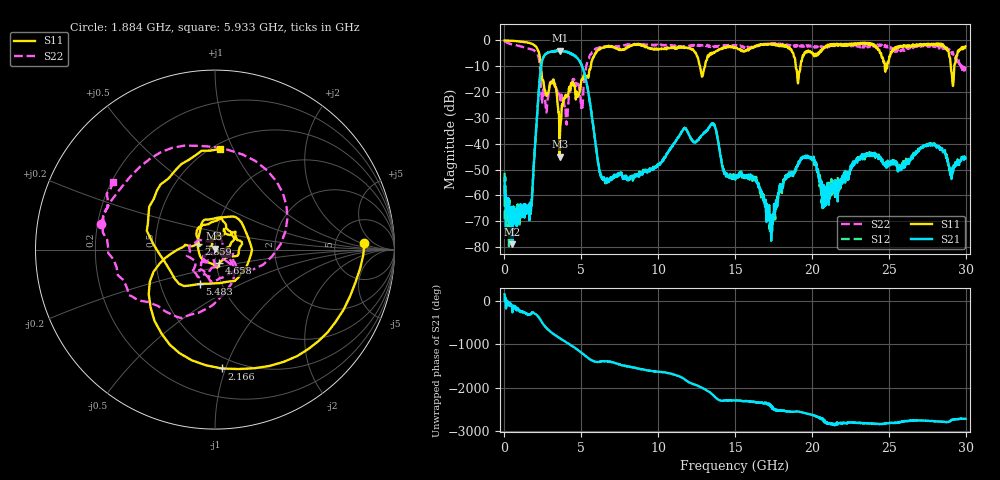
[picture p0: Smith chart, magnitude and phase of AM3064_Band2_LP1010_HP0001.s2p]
# Hz S DB R 50.0
!freq dBS11 angS11 dBS21 angS21 dBS12 angS12 dBS22 angS22
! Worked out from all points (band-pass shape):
!   1600 points, 10 MHz to 29.98 GHz, reference 50 ohm
!   highest |S21| = -3.93 dB at 3.59 GHz (marker M1); lowest = -79.0 dB at 516.1 MHz (marker M2)
!   |S21| within 3 dB of the highest: 2.507 GHz to 4.753 GHz (2.246 GHz wide, 61.9 % of centre)
!   lowest |S11| = -45.0 dB at 3.59 GHz (marker M3), VSWR 1.01, Z = 49.7 + j0.497 ohm
!   |S11| at or under -10 dB: 2.374 GHz to 5.616 GHz (3.242 GHz wide, 81.2 % of centre); 12.72 GHz to 13.05 GHz (328.4 MHz wide, 2.55 % of centre); 18.95 GHz to 19.25 GHz (304.2 MHz wide, 1.59 % of centre)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
!   |S22| runs from -32.6 to -0.3 dB; largest |S21 - S12| = 0.021
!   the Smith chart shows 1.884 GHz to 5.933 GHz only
!   S11 on the Smith chart (normalised r, x): 1.884 GHz: 10, +3; 2.166 GHz: 0.41, -0.97; 2.859 GHz: 0.83, +0.05; 4.658 GHz: 1.04, -0.15; 5.483 GHz: 0.79, -0.32; 5.933 GHz: 0.55, +0.89
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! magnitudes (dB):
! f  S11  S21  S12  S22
! 10 MHz  0.0  -53.4  -51.3  -0.3
! 516.1 MHz  -0.2  -79.0  -64.4  -1.5
! 1.622 GHz  -1.0  -69.7  -66.0  -3.3
! 1.884 GHz  -1.6  -50.7  -50.6  -3.7
! 2.166 GHz  -3.6  -25.1  -25.1  -5.5
! 2.859 GHz  -20.2  -4.6  -4.7  -21.2
! 3.59 GHz  -45.0  -3.9  -4.0  -21.5
! 4.658 GHz  -22.2  -6.4  -6.3  -17.1
! 5.015 GHz  -15.3  -9.6  -9.4  -24.3
! 5.483 GHz  -13.6  -21.0  -21.0  -7.1
! 5.933 GHz  -5.0  -40.4  -40.4  -3.3
! 6.664 GHz  -2.2  -53.3  -55.2  -2.5
! 10 GHz  -3.4  -48.0  -47.9  -1.8
! 13.54 GHz  -5.1  -32.4  -32.1  -2.5
! 15 GHz  -2.6  -53.9  -52.3  -1.9
! 17.39 GHz  -1.6  -69.3  -70.9  -1.3
! 19.99 GHz  -4.6  -45.7  -46.4  -2.0
! 20.82 GHz  -2.8  -62.4  -56.8  -2.3
! 25 GHz  -7.9  -47.8  -47.8  -2.3
! 28.39 GHz  -1.3  -42.1  -42.4  -3.1
! 29.18 GHz  -17.6  -50.9  -48.5  -4.8
! 29.98 GHz  -2.3  -45.8  -44.9  -10.2
